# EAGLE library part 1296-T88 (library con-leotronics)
1.27mm SINGLE ROW FEMALE SOCKET Source: http://www.leotronics.co.uk/Conexcon/Data%20Sheets/sec.%20A/1296ing.pdf
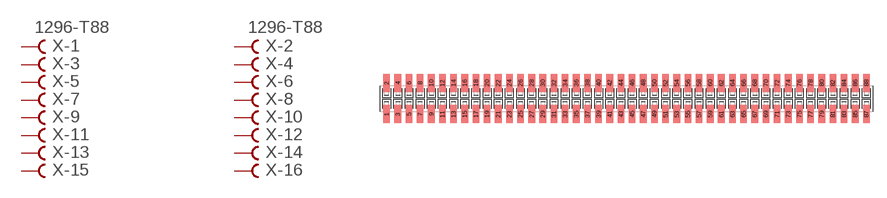
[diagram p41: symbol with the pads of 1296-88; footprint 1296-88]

Designator prefix X; gates -1=FVAL -2=FVAL -3=F -4=F -5=F -6=F -7=F -8=F -9=F -10=F -11=F -12=F -13=F -14=F -15=F -16=F -17=F -18=F -19=F -20=F -21=F -22=F -23=F -24=F -25=F -26=F -27=F -28=F -29=F -30=F -31=F -32=F -33=F -34=F -35=F -36=F -37=F -38=F -39=F -40=F -41=F -42=F -43=F -44=F -45=F -46=F -47=F -48=F -49=F -50=F -51=F -52=F -53=F -54=F -55=F -56=F -57=F -58=F -59=F -60=F -61=F -62=F -63=F -64=F -65=F -66=F -67=F -68=F -69=F -70=F -71=F -72=F -73=F -74=F -75=F -76=F -77=F -78=F -79=F -80=F -81=F -82=F -83=F -84=F -85=F -86=F -87=F -88=F

## 1296-T88 (OC_FARNELL: unknown; OC_NEWARK: unknown)  [1296-88]
1  -1:B  pas
2  -2:B  pas
3  -3:B  pas
4  -4:B  pas
5  -5:B  pas
6  -6:B  pas
7  -7:B  pas
8  -8:B  pas
9  -9:B  pas
10  -10:B  pas
11  -11:B  pas
12  -12:B  pas
13  -13:B  pas
14  -14:B  pas
15  -15:B  pas
16  -16:B  pas
17  -17:B  pas
18  -18:B  pas
19  -19:B  pas
20  -20:B  pas
21  -21:B  pas
22  -22:B  pas
23  -23:B  pas
24  -24:B  pas
25  -25:B  pas
26  -26:B  pas
27  -27:B  pas
28  -28:B  pas
29  -29:B  pas
30  -30:B  pas
31  -31:B  pas
32  -32:B  pas
33  -33:B  pas
34  -34:B  pas
35  -35:B  pas
36  -36:B  pas
37  -37:B  pas
38  -38:B  pas
39  -39:B  pas
40  -40:B  pas
41  -41:B  pas
42  -42:B  pas
43  -43:B  pas
44  -44:B  pas
45  -45:B  pas
46  -46:B  pas
47  -47:B  pas
48  -48:B  pas
49  -49:B  pas
50  -50:B  pas
51  -51:B  pas
52  -52:B  pas
53  -53:B  pas
54  -54:B  pas
55  -55:B  pas
56  -56:B  pas
57  -57:B  pas
58  -58:B  pas
59  -59:B  pas
60  -60:B  pas
61  -61:B  pas
62  -62:B  pas
63  -63:B  pas
64  -64:B  pas
65  -65:B  pas
66  -66:B  pas
67  -67:B  pas
68  -68:B  pas
69  -69:B  pas
70  -70:B  pas
71  -71:B  pas
72  -72:B  pas
73  -73:B  pas
74  -74:B  pas
75  -75:B  pas
76  -76:B  pas
77  -77:B  pas
78  -78:B  pas
79  -79:B  pas
80  -80:B  pas
81  -81:B  pas
82  -82:B  pas
83  -83:B  pas
84  -84:B  pas
85  -85:B  pas
86  -86:B  pas
87  -87:B  pas
88  -88:B  pas

## Footprint 1296-88 (pad centres in mm)
1.27mm SINGLE ROW FEMALE SOCKET Source: http://www.leotronics.co.uk/Conexcon/Data%20Sheets/sec.%20A/1296ing.pdf
smd 0.76 x 2.05: 1 -27.305,-1.78; 2 -27.305,1.78; 3 -26.035,-1.78; 4 -26.035,1.78; 5 -24.765,-1.78; 6 -24.765,1.78; 7 -23.495,-1.78; 8 -23.495,1.78; 9 -22.225,-1.78; 10 -22.225,1.78; 11 -20.955,-1.78; 12 -20.955,1.78; 13 -19.685,-1.78; 14 -19.685,1.78; 15 -18.415,-1.78; 16 -18.415,1.78; 17 -17.145,-1.78; 18 -17.145,1.78; 19 -15.875,-1.78; 20 -15.875,1.78; 21 -14.605,-1.78; 22 -14.605,1.78; 23 -13.335,-1.78; 24 -13.335,1.78; 25 -12.065,-1.78; 26 -12.065,1.78; 27 -10.795,-1.78; 28 -10.795,1.78; 29 -9.525,-1.78; 30 -9.525,1.78; 31 -8.255,-1.78; 32 -8.255,1.78; 33 -6.985,-1.78; 34 -6.985,1.78; 35 -5.715,-1.78; 36 -5.715,1.78; 37 -4.445,-1.78; 38 -4.445,1.78; 39 -3.175,-1.78; 40 -3.175,1.78; 41 -1.905,-1.78; 42 -1.905,1.78; 43 -0.635,-1.78; 44 -0.635,1.78; 45 0.635,-1.78; 46 0.635,1.78; 47 1.905,-1.78; 48 1.905,1.78; 49 3.175,-1.78; 50 3.175,1.78; 51 4.445,-1.78; 52 4.445,1.78; 53 5.715,-1.78; 54 5.715,1.78; 55 6.985,-1.78; 56 6.985,1.78; 57 8.255,-1.78; 58 8.255,1.78; 59 9.525,-1.78; 60 9.525,1.78; 61 10.795,-1.78; 62 10.795,1.78; 63 12.065,-1.78; 64 12.065,1.78; 65 13.335,-1.78; 66 13.335,1.78; 67 14.605,-1.78; 68 14.605,1.78; 69 15.875,-1.78; 70 15.875,1.78; 71 17.145,-1.78; 72 17.145,1.78; 73 18.415,-1.78; 74 18.415,1.78; 75 19.685,-1.78; 76 19.685,1.78; 77 20.955,-1.78; 78 20.955,1.78; 79 22.225,-1.78; 80 22.225,1.78; 81 23.495,-1.78; 82 23.495,1.78; 83 24.765,-1.78; 84 24.765,1.78; 85 26.035,-1.78; 86 26.035,1.78; 87 27.305,-1.78; 88 27.305,1.78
